{attribute 'qualified_only'}
VAR_GLOBAL
	AXISX: AXIS_REF;
		
	// SDO Write
	SdoWriteExe  :BOOL;//SDO Write Execution
	SdoWriteValue  :DINT;//Buffer data for writing
	SdoWriteIndex  :WORD;// SDO Index
	SdoWriteSubIndex  :BYTE;// SDO Sub-index
	SdoWriteSrcBuf  :PVOID;// Reference address of buffer data
	SdoWriteBufLen  :UDINT;//Write data length
	SdoWriteError  :BOOL;//SDO Write Error bit
	SdoWriteErrId  :UDINT;//SDO Write Error ID
	
	// SDO Read
	SdoReadExe	:BOOL;//SDO Read Execution
	SdoReadValue  :DINT;//Buffer data for reading
	SdoReadIndex  :WORD;//SDO Index
	SdoReadSubIndex :BYTE;//SDO Sub-Index
	SdoReadSrcBuf  :PVOID;//Reference address of buffer data
	SdoReadBufLen  :UDINT;//Read Buffer Data Length
	SdoReadError  :BOOL;//SDO Read Error
	SdoReadErrId  :UDINT;//SDO Read ErrorID
END_VAR
